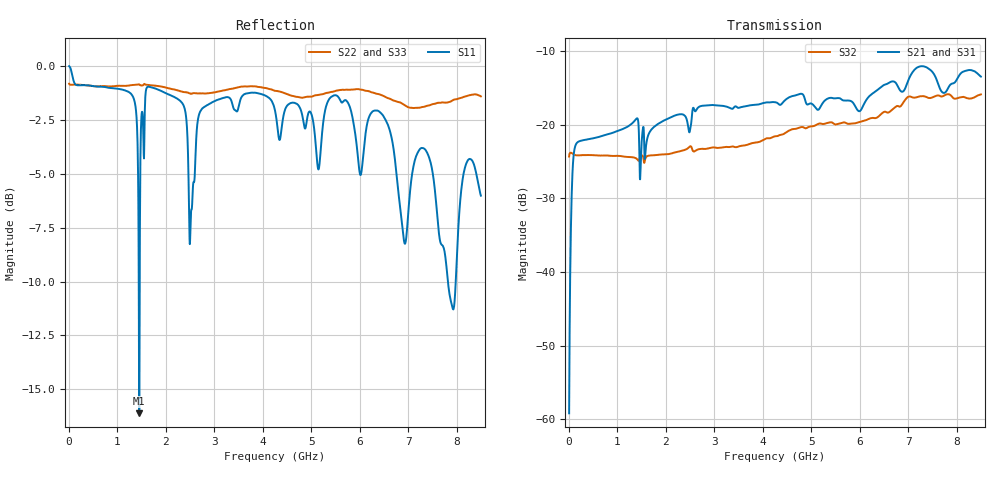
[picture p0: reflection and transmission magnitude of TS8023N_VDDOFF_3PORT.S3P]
!Agilent Technologies,E5071C,MY46522130,B.12.04
!Date: Thu Jul 17 20:31:59 2025
!Data & Calibration Information:
!Freq	S11:SOLT3(ON)	S13:SOLT3(ON)	S14:SOLT3(ON)
!	S31:SOLT3(ON)	S33:SOLT3(ON)	S34:SOLT3(ON)
!	S41:SOLT3(ON)	S43:SOLT3(ON)	S44:SOLT3(ON)
!PortZ  Port1:50+j0  Port3:50+j0  Port4:50+j0
!Above PortZ is port z conversion or system Z0 setting when saving the data.
!When reading, reference impedance value at option line is always used.
# Hz S dB R 50
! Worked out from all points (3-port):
!   1601 points, 10 MHz to 8.5 GHz, reference 50 ohm
!   strongest paths, dB at 10 MHz, 2.132 GHz, 4.255 GHz, 6.378 GHz, 8.5 GHz:
!     S21: -59.2, -18.9, -16.9, -15.2, -13.5
!     S31: -59.3, -19.0, -17.0, -15.0, -13.1
!     S32: -24.3, -23.9, -21.6, -18.9, -15.9
!   lowest |S11| = -16.1 dB at 1.453 GHz (marker M1), VSWR 1.37, Z = 63.8 + j11.3 ohm
!   |S11| at or under -10 dB: 1.446 GHz to 1.466 GHz (19.95 MHz wide, 1.37 % of centre); 7.82 GHz to 7.981 GHz (161.5 MHz wide, 2.04 % of centre)
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1e7  0.00 163.0  -59.40 -174.9  -59.34 -173.0
     -59.19 -174.5  -0.81 178.6  -24.32 17.9
     -59.31 -173.4  -24.32 17.9  -0.81 178.6
5.775625e7  -0.24 72.7  -30.78 128.3  -30.82 128.5
            -30.79 128.1  -0.86 179.1  -23.82 1.7
            -30.83 128.4  -23.83 1.7  -0.86 179.2
1.002062e8  -0.66 -11.4  -24.33 85.6  -24.36 85.8
            -24.36 85.7  -0.86 178.8  -24.00 -0.4
            -24.39 85.8  -24.01 -0.3  -0.86 178.8
1.744938e8  -0.88 -89.5  -22.44 48.2  -22.48 48.2
            -22.44 48.4  -0.85 178.1  -24.14 -0.7
            -22.48 48.5  -24.17 -0.8  -0.86 177.9
4.451125e8  -0.90 -150.8  -21.95 22.3  -22.02 22.4
            -21.92 22.4  -0.91 174.5  -24.16 -1.9
            -22.00 22.5  -24.13 -1.9  -0.90 174.5
1.272888e9  -1.25 166.6  -20.01 10.9  -20.01 11.3
            -20.01 11.0  -0.88 162.6  -24.39 -6.1
            -20.00 11.4  -24.39 -6.1  -0.88 163.1
1.4533e9  -16.12 33.6  -22.22 -29.8  -22.37 -29.9
          -22.23 -29.9  -0.84 161.0  -24.81 -3.1
          -22.39 -29.9  -24.83 -3.0  -0.83 160.9
1.676162e9  -0.96 177.3  -20.95 19.8  -20.94 19.8
            -20.94 19.8  -0.88 159.1  -24.20 -4.2
            -20.94 19.8  -24.17 -4.4  -0.88 158.9
4.255e9  -2.05 88.8  -16.93 -15.9  -16.94 -16.5
         -16.94 -15.5  -1.14 130.8  -21.55 -13.0
         -16.98 -16.2  -21.57 -13.2  -1.15 129.1
8.5e9  -6.01 42.2  -13.38 -55.2  -13.05 -56.3
       -13.46 -54.8  -1.40 76.1  -15.87 -62.8
       -13.06 -56.2  -15.88 -63.4  -1.57 72.1
